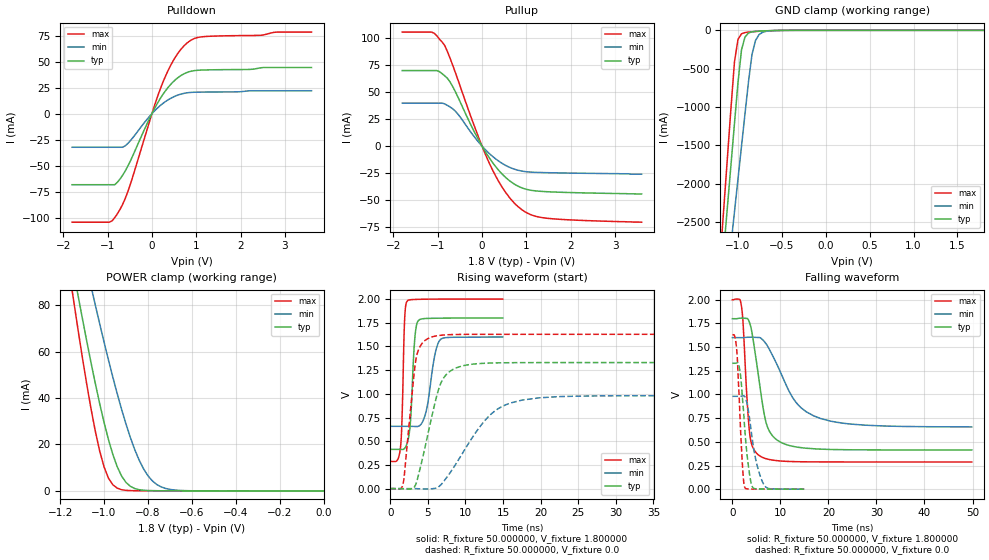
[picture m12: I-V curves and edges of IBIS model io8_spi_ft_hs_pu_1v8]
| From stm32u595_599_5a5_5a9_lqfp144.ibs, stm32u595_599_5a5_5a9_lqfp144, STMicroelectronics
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|   Model io8_spi_ft_hs_pu_1v8
[Model]  io8_spi_ft_hs_pu_1v8
Model_type I/O
Polarity   Non-Inverting
Enable   Active-Low
Vinl =   0.540000V
Vinh =   1.260000V
Vmeas =  0.900000V
Cref =   50.000000pF
Rref =   100.000000M
Vref =   0.0V
C_comp   3.338500pF   3.332300pF   3.378900pF
[Temperature Range]   25.000000   0.140000k   -40.000000
[Pullup Reference]   1.800000V   1.600000V   2.000000V
[Pulldown Reference]   0.0V   0.0V   0.0V
[POWER Clamp Reference]   1.800000V   1.600000V   2.000000V
[GND Clamp Reference]   0.0V   0.0V   0.0V
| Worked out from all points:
|   slope of the pulldown table from 0 to 0.27 V, typ, clamps not added: 13.6 ohm
|   slope of the pullup table from 0 to 0.27 V, typ, clamps not added: 15.9 ohm
|   GND clamp passes 1 mA (typ) near -0.51 V on its own axis
|   POWER clamp passes 1 mA (typ) near -0.86 V on its own axis
|   rising waveform, R_fixture 50.000000, V_fixture 1.800000: 20-80 % time 534ps typ, 1.08ns min, 335ps max; typ from 0.414 V to 1.8 V
|   rising waveform, R_fixture 50.000000, V_fixture 0.0: 20-80 % time 2.37ns typ, 5.18ns min, 1.21ns max; typ from 0 V to 1.33 V
|   falling waveform, R_fixture 50.000000, V_fixture 1.800000: 20-80 % time 2.6ns typ, 6.29ns min, 1.18ns max; typ from 1.8 V to 0.414 V
|   falling waveform, R_fixture 50.000000, V_fixture 0.0: 20-80 % time 1.33ns typ, 1.97ns min, 906ps max; typ from 1.33 V to 0 V
[Pulldown]
|Voltage   I(typ)   I(min)   I(max)
-1.8V     -68.38mA   -32.32mA   -104.4mA
-960mV    -68.38mA   -32.32mA   -104.4mA
-780mV    -66.07mA   -32.32mA   -96.42mA
-660mV    -59.2mA    -32.31mA   -87.22mA
-540mV    -50.22mA   -28.51mA   -74.66mA
0V        0A         0A         0A
240mV     18.04mA    9.599mA    29.41mA
480mV     30.68mA    16.02mA    50.95mA
780mV     39.47mA    19.98mA    67.56mA
960mV     41.44mA    20.62mA    72.37mA
1.14V     41.98mA    20.78mA    74.01mA
3.6V      44.42mA    22.05mA    78.5mA
[Pullup]
|Voltage   I(typ)   I(min)   I(max)
-1.8V     70.05mA    39.89mA    105.7mA
-1.14V    70.05mA    39.89mA    105.7mA
-960mV    69.07mA    39.89mA    99.14mA
-840mV    65.1mA     39.14mA    93.13mA
-600mV    50.32mA    32.31mA    68mA
-180mV    13.77mA    8.913mA    19.32mA
180mV     -11.9mA    -7.442mA   -17.26mA
480mV     -26.98mA   -16.65mA   -39.76mA
840mV     -37.65mA   -22.63mA   -57.07mA
1.08V     -40.74mA   -24.01mA   -63.22mA
1.44V     -42.19mA   -24.58mA   -66.73mA
3.6V      -44.3mA    -26mA      -70.5mA
[GND_clamp]
|Voltage   I(typ)   I(min)   I(max)
-1.8V     -9.908A    -9.683A    -9.994A
-1.2V     -3.383A    -4.084A    -2.934A
-1.16V    -2.841A    -3.655A    -2.294A
-1.12V    -2.299A    -3.226A    -1.656A
-1.04V    -1.218A    -2.369A    -414.2mA
-1V       -684.7mA   -1.941A    -119.2mA
-960mV    -257.2mA   -1.514A    -45.66mA
-920mV    -87.03mA   -1.089A    -28.93mA
-840mV    -19.35mA   -312.8mA   -18.96mA
-800mV    -13.55mA   -132.4mA   -15.49mA
-720mV    -8.042mA   -25.66mA   -9.49mA
1.8V      0A         13.64nA    0A
[POWER_clamp]
|Voltage   I(typ)   I(min)   I(max)
-1.8V     470.9mA    433.7mA    554.6mA
-1.14V    95.28mA    122.7mA    82.88mA
-1.12V    85mA       114mA      70.34mA
-1.06V    55.55mA    88.43mA    35.73mA
-1.04V    46.38mA    80.17mA    25.83mA
-1V       29.54mA    64.14mA    10.37mA
-940mV    10.43mA    41.88mA    1.177mA
-900mV    3.66mA     28.79mA    250.5uA
-840mV    527.2uA    13.26mA    95.12uA
-800mV    153.8uA    6.55mA     88.66uA
-740mV    59.96uA    1.741mA    70.48uA
0V        0A         18.18nA    0A
[Ramp]
| variable   typ   min   max
dV/dt_r  0.79756/2.36245n   0.58806/5.17433n   0.97651/1.21224n
dV/dt_f  0.83131/2.59353n   0.56514/6.27963n   1.02742/1.18003n
R_load = 50.000000
[Rising Waveform]
R_fixture= 50.000000
V_fixture= 1.800000
V_fixture_min= 1.600000
V_fixture_max= 2.000000
|time   V(typ)   V(min)   V(max)
0s        414.5mV    657.5mV    287.6mV
1.351ns   413.8mV    657.5mV    428.6mV
1.562ns   412.8mV    657.5mV    738.3mV
1.892ns   423.3mV    657.6mV    1.751V
2.222ns   474.8mV    657.5mV    1.976V
2.673ns   692.9mV    657.4mV    1.993V
3.303ns   1.619V     655.8mV    1.996V
3.724ns   1.771V     657.3mV    1.997V
6.547ns   1.798V     1.562V     1.999V
14.95ns   1.8V       1.6V       2V
[Rising Waveform]
R_fixture= 50.000000
V_fixture= 0.0
V_fixture_min= 0.0
V_fixture_max= 0.0
|time   V(typ)   V(min)   V(max)
0s        426.4uV    509.7uV    392.8uV
1.702ns   -1.704mV   507.6uV    50.65mV
3.403ns   45.45mV    239.7uV    1.36V
4.004ns   224.4mV    -2.441mV   1.505V
5.205ns   646.6mV    -2.977mV   1.59V
6.507ns   1.066V     24.65mV    1.616V
7.808ns   1.229V     150.7mV    1.624V
12.61ns   1.323V     721.1mV    1.628V
16.02ns   1.328V     903.9mV    1.628V
49.85ns   1.33V      980.7mV    1.628V
[Falling Waveform]
R_fixture= 50.000000
V_fixture= 1.800000
V_fixture_min= 1.600000
V_fixture_max= 2.000000
|time   V(typ)   V(min)   V(max)
0s        1.8V       1.6V       2V
1.902ns   1.806V     1.6V       1.929V
2.202ns   1.806V     1.6V       1.775V
3.604ns   1.755V     1.605V     587.7mV
5.606ns   1.134V     1.602V     355mV
6.907ns   725.3mV    1.542V     323.6mV
8.408ns   560.8mV    1.408V     306.9mV
12.71ns   451.5mV    955.2mV    291.6mV
17.02ns   426.9mV    772.4mV    288.4mV
49.85ns   414.5mV    657.5mV    287.6mV
[Falling Waveform]
R_fixture= 50.000000
V_fixture= 0.0
V_fixture_min= 0.0
V_fixture_max= 0.0
|time   V(typ)   V(min)   V(max)
0s        1.33V      980.7mV    1.628V
900.9ps   1.333V     980.7mV    1.476V
1.742ns   1.183V     981.3mV    587.7mV
2.252ns   868.3mV    986.4mV    137.4mV
2.613ns   612.5mV    975mV      16.09mV
3.273ns   271.5mV    847.2mV    3.205mV
4.024ns   43.28mV    574.7mV    1.782mV
5.105ns   3.738mV    261.7mV    1.179mV
6.517ns   1.696mV    52.38mV    839.6uV
14.95ns   426.4uV    509.7uV    392.8uV
